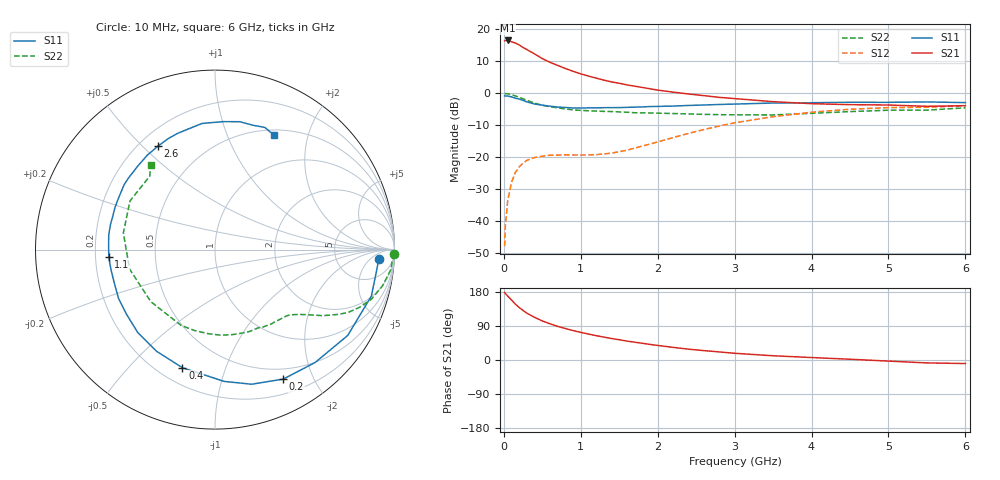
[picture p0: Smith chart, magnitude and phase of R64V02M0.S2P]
! SIEMENS Small Signal Semiconductors
! BFR193
! Si NPN RF Bipolar Junction Transistor in SOT23
! VCE = 4 V  IC = 2 mA
! Common Emitter S-Parameters:  May  1996
# GHz  S  MA  R  50
!  f  S11  S21  S12  S22
! GHz  MAG  ANG  MAG  ANG  MAG  ANG  MAG  ANG
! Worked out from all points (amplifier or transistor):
!   36 points, 10 MHz to 6 GHz, reference 50 ohm
!   highest |S21| = 16.5 dB at 50 MHz (marker M1)
!   |S21| within 3 dB of that: start of sweep to 310.7 MHz
!   unconditionally stable (mu >= 1): 1.149 GHz to 2.047 GHz
!   at 250 MHz: K = 0.23, MSG = 18.1 dB, |S12| = -21.8 dB
!   at 1.4 GHz: K = 1.11, MAG = 9.1 dB, |S12| = -18.7 dB
!   at 6 GHz: K = 0.99, MSG = 0.0 dB, |S12| = -3.9 dB
!   S11 on the Smith chart (normalised r, x): 10 MHz: 16, -10; 200 MHz: 0.37, -1.60; 400 MHz: 0.29, -0.72; 1.1 GHz: 0.26, -0.03; 2.6 GHz: 0.27, +0.56; 6 GHz: 0.57, +1.49
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0.01  0.9135 -3.3  6.603 178.2  0.0041 86.8  0.9975 -1.3
0.02  0.909 -6.5  6.669 175.4  0.0086 86.4  0.9915 -2.5
0.05  0.9089 -16.6  6.709 168.8  0.021 80.7  0.9861 -6.5
0.1  0.8807 -32.9  6.401 158.3  0.0409 72.2  0.9545 -12.3
0.15  0.8408 -48.4  6.114 147.3  0.0579 64.2  0.9141 -17.6
0.2  0.8156 -62.2  5.704 138.5  0.071 57.7  0.8669 -21.8
0.25  0.7773 -74.8  5.203 130.6  0.0814 51.7  0.821 -25.2
0.3  0.7359 -86.1  4.829 123.5  0.09 47.6  0.7786 -27.6
0.4  0.6827 -105.4  4.134 112.5  0.0994 40.6  0.7046 -31.5
0.5  0.6534 -119.9  3.497 103.1  0.1043 36.3  0.6515 -34.0
0.6  0.6314 -133.0  3.057 95.5  0.1081 33.8  0.619 -35.8
0.7  0.6103 -144.1  2.732 88.7  0.1087 32.6  0.5935 -37.5
0.9  0.5913 -161.4  2.216 77.7  0.1091 33.8  0.5527 -41.2
1.1  0.5933 -175.9  1.864 68.5  0.1094 37.7  0.5351 -45.5
1.3  0.5977 172.1  1.61 60.5  0.1133 43.8  0.523 -50.0
1.6  0.6046 157.2  1.356 49.9  0.1294 54.1  0.5076 -58.2
2.2  0.6333 133.1  1.045 33.3  0.2039 63.8  0.4839 -78.1
2.6  0.6581 118.9  0.922 24.8  0.2722 62.0  0.4699 -94.7
3.5  0.7065 95.9  0.742 11.2  0.4325 46.9  0.4605 -140.9
4.5  0.7258 79.0  0.666 2.0  0.5647 25.9  0.519 169.7
5.5  0.7352 67.8  0.628 -7.7  0.6068 6.6  0.5474 131.6
6  0.7171 62.6  0.643 -9.3  0.6405 1.3  0.5939 127.1
